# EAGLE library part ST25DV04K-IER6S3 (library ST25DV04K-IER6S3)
STMICROELECTRONICS - ST25DV04K-IER6S3 - RFID/NFC IC, 13.553 MHz to 13.567 MHz, Read, Write, 4Kbit, I2C, 1.8 V to 5.5 V, SOIC-8 Source: Datasheet
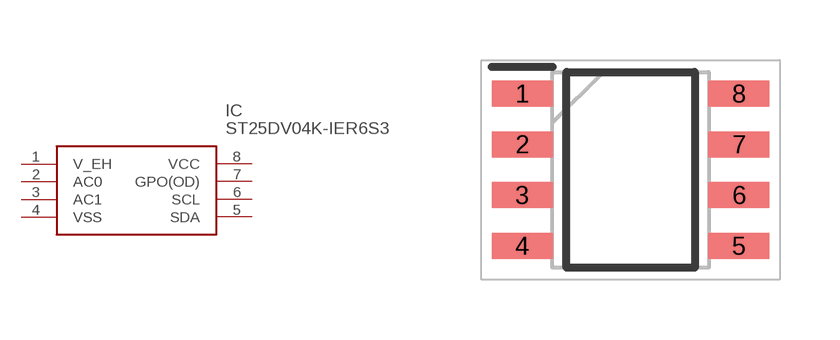
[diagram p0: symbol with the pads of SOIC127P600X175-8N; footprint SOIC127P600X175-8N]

Designator prefix IC

## ST25DV04K-IER6S3 (Arrow_Part_Number: ST25DV04K-IER6S3; Arrow_Price-Stock: https://www.arrow.com/en/products/st25dv04k-ier6s3/stmicroelectronics?region=nac; Description: STMICROELECTRONICS - ST25DV04K-IER6S3 - RFID/NFC IC, 13.553 MHz to 13.567 MHz, Read, Write, 4Kbit, I2C, 1.8 V to 5.5 V, SOIC-8; Height: 1.75mm; Manufacturer_Name: STMicroelectronics; Manufacturer_Part_Number: ST25DV04K-IER6S3; Mouser_Part_Number: 511-ST25DV04K-IER6S3; Mouser_Price-Stock: https://www.mouser.co.uk/ProductDetail/STMicroelectronics/ST25DV04K-IER6S3?qs=xjeEZJU9OeNdtP1j9447OQ%3D%3D)  [SOIC127P600X175-8N]
1  V_EH
2  AC0
3  AC1
4  VSS
5  SDA
6  SCL
7  GPO(OD)
8  VCC

## Footprint SOIC127P600X175-8N (pad centres in mm)
SO8N &ndash; 8-lead plastic small outline, 150 mils body width
smd 1.525 x 0.65: 1 -2.712,1.905; 2 -2.712,0.635; 3 -2.712,-0.635; 4 -2.712,-1.905; 5 2.712,-1.905; 6 2.712,-0.635; 7 2.712,0.635; 8 2.712,1.905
